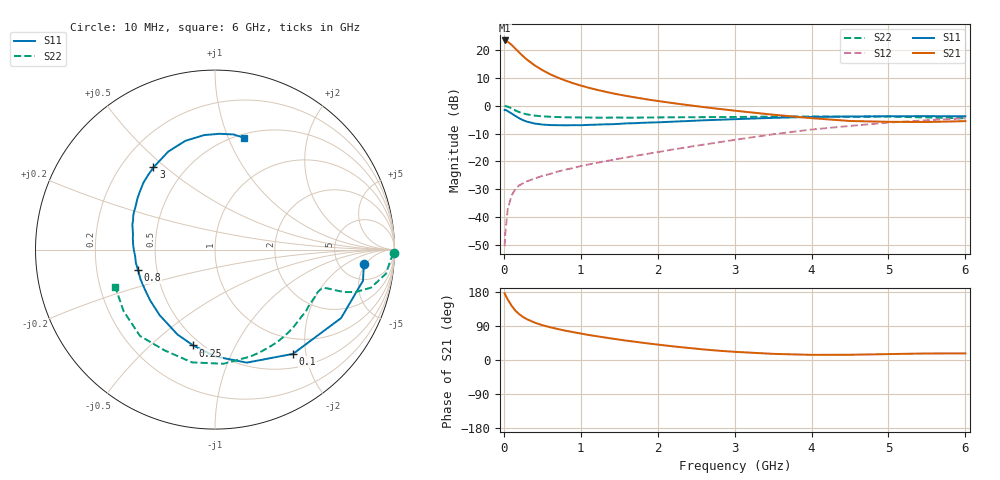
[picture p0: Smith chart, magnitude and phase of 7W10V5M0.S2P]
! Infineon Technologies  Discrete & RF Semiconductors
! BFS17W
! Si NPN RF Bipolar Junction Transistor in SOT323
! VCE = 10 V  IC = 5 mA
! Common Emitter S-Parameters:  August  1999
# GHz  S  MA  R  50
!  f  S11  S21  S12  S22
! GHz  MAG  ANG  MAG  ANG  MAG  ANG  MAG  ANG
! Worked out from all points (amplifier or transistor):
!   36 points, 10 MHz to 6 GHz, reference 50 ohm
!   highest |S21| = 23.4 dB at 10 MHz (marker M1)
!   |S21| within 3 dB of that: start of sweep to 152.9 MHz
!   unconditionally stable (mu >= 1): 590.7 MHz to 2.287 GHz; 5.325 GHz to end of sweep
!   at 250 MHz: K = 0.57, MSG = 22.8 dB, |S12| = -27.9 dB
!   at 1.4 GHz: K = 1.20, MAG = 9.3 dB, |S12| = -19.6 dB
!   at 6 GHz: K = 1.05, MAG = -1.9 dB, |S12| = -4.5 dB
!   S11 on the Smith chart (normalised r, x): 10 MHz: 8.50, -4.62; 100 MHz: 0.72, -1.77; 250 MHz: 0.45, -0.69; 800 MHz: 0.39, -0.11; 3 GHz: 0.33, +0.46; 6 GHz: 0.54, +1.15
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0.01  0.8339 -5.7  14.84 176.1  0.003 83.6  0.9963 -1.2
0.02  0.8424 -11.9  14.83 171.6  0.0052 92.4  0.98 -3.3
0.05  0.7993 -28.5  14.12 159.9  0.0136 76.8  0.9623 -8.0
0.1  0.7255 -53.2  12.4 143.5  0.0243 66.1  0.8946 -13.7
0.15  0.6542 -74.3  10.6 130.3  0.0317 58.7  0.8205 -16.7
0.2  0.595 -90.0  9.031 120.9  0.0371 54.9  0.7669 -18.0
0.25  0.5478 -102.8  7.738 113.5  0.0404 51.4  0.7263 -18.5
0.3  0.5173 -113.8  6.736 107.7  0.0438 51.6  0.6992 -18.7
0.4  0.478 -130.3  5.307 98.7  0.0492 51.7  0.6634 -19.0
0.5  0.4588 -142.1  4.357 92.0  0.0548 53.0  0.6445 -19.4
0.6  0.4487 -151.4  3.679 86.5  0.0595 55.0  0.6327 -20.1
0.8  0.4435 -164.9  2.831 77.4  0.0709 58.2  0.6192 -22.6
0.9  0.4472 -170.4  2.533 73.6  0.0759 60.0  0.6152 -24.0
1.1  0.4519 -179.7  2.107 66.1  0.088 62.4  0.6124 -27.5
1.3  0.4619 172.4  1.807 59.8  0.0999 64.4  0.6093 -31.3
1.6  0.4813 163.0  1.49 50.9  0.1181 67.3  0.6098 -37.4
2.2  0.5172 146.8  1.112 36.0  0.1635 71.3  0.6184 -51.4
3  0.5722 126.8  0.814 21.6  0.2432 71.7  0.6273 -71.6
3.5  0.605 115.5  0.689 16.2  0.3067 69.0  0.6378 -85.7
4.5  0.6408 95.4  0.531 13.8  0.433 57.6  0.6278 -116.5
5.5  0.6498 80.9  0.509 17.2  0.5485 44.2  0.6142 -146.0
6  0.6434 75.2  0.528 17.4  0.5937 37.4  0.5935 -159.3
